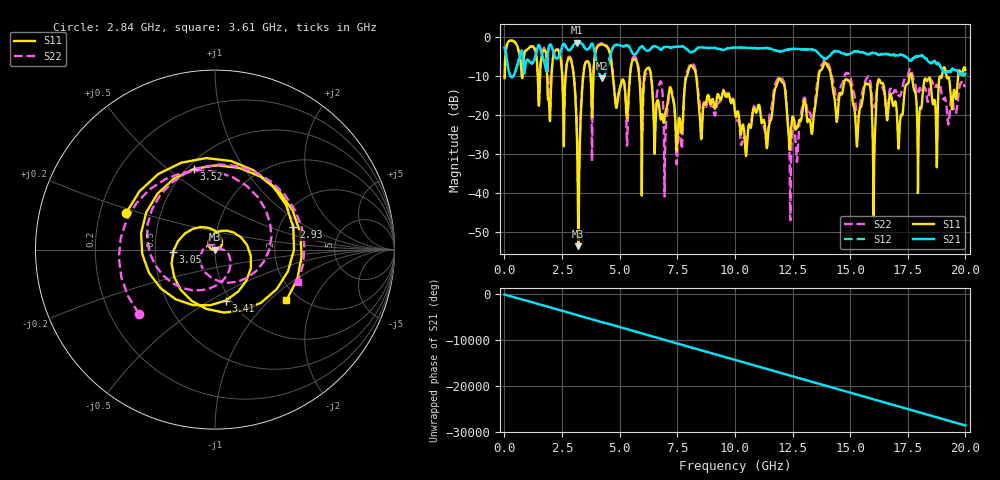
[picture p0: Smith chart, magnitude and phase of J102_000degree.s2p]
!Keysight Technologies,N5222A,MY51421036,A.10.65.16
!Date: Friday, March 31, 2023 14:53:39
!Correction: S11(Full 2 Port(1,2))
!S21(Full 2 Port(1,2))
!S12(Full 2 Port(1,2))
!S22(Full 2 Port(1,2))
!S2P File: Measurements: S11, S21, S12, S22:
# Hz S  dB  R 50
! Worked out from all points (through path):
!   2000 points, 10 MHz to 20 GHz, reference 50 ohm
!   highest |S21| = -1.46 dB at 3.16 GHz (marker M1); lowest = -10.6 dB at 4.24 GHz (marker M2)
!   group delay of S21, straight-line fit = 3.98 ns
!   lowest |S11| = -53.7 dB at 3.21 GHz (marker M3), VSWR 1.00, Z = 50.2 + j0.019 ohm
!   |S11| at or under -10 dB: 6.362 GHz to 7.919 GHz (1.557 GHz wide, 21.8 % of centre); 8.32 GHz to 13.64 GHz (5.321 GHz wide, 48.5 % of centre); 14.17 GHz to 17.59 GHz (3.412 GHz wide, 21.5 % of centre)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
!   |S22| runs from -47.1 to -0.9 dB; largest |S21 - S12| = 0.02
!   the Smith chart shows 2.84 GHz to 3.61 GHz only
!   S11 on the Smith chart (normalised r, x): 2.84 GHz: 0.31, +0.18; 2.93 GHz: 2.38, +0.75; 3.05 GHz: 0.62, -0.01; 3.41 GHz: 0.95, -0.59; 3.52 GHz: 0.54, +0.62; 3.61 GHz: 1.72, -1.28
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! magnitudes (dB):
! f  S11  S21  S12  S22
! 10 MHz  -10.6  -2.7  -2.6  -10.5
! 2.84 GHz  -5.4  -3.5  -3.4  -5.1
! 2.93 GHz  -6.9  -2.8  -2.7  -6.6
! 3.05 GHz  -12.6  -1.7  -1.7  -12.4
! 3.16 GHz  -28.9  -1.5  -1.4  -27.4
! 3.21 GHz  -53.7  -1.5  -1.4  -33.6
! 3.35 GHz  -15.9  -1.7  -1.7  -15.0
! 3.41 GHz  -10.7  -2.1  -2.0  -10.4
! 3.52 GHz  -6.7  -3.1  -3.0  -6.5
! 3.61 GHz  -6.2  -3.2  -3.2  -6.1
! 4.24 GHz  -1.9  -10.6  -10.6  -1.6
! 5.31 GHz  -20.7  -2.2  -2.1  -26.4
! 5.62 GHz  -5.7  -4.5  -4.5  -5.0
! 6.68 GHz  -16.6  -2.8  -2.7  -12.9
! 7.53 GHz  -23.6  -2.5  -2.5  -27.4
! 8.1 GHz  -7.3  -4.0  -4.0  -6.8
! 8.53 GHz  -26.0  -2.8  -2.7  -20.4
! 10.01 GHz  -19.6  -2.7  -2.7  -19.3
! 13.34 GHz  -24.9  -3.3  -3.2  -21.1
! 13.92 GHz  -6.6  -5.7  -5.6  -5.9
! 16.67 GHz  -17.5  -4.6  -4.4  -15.8
! 20 GHz  -8.5  -9.4  -9.0  -12.7
